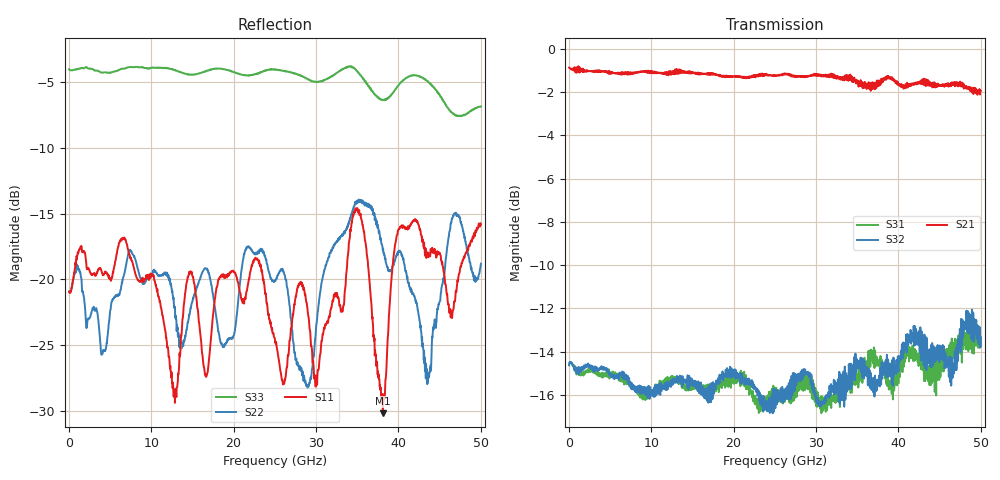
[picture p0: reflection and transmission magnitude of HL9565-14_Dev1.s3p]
! 1/5/2021 8:28:36 AM
! H:\PRODUCTION_DATA\TEMP_S3P.S3P
! CHANNEL.1
! TR.MEASUREMENT
! CORRECTED.DATA
# GHZ S RI R 50.0
! FREQ.GHZ  S11RE  S11IM  S12RE  S12IM  S13RE  S13IM
!  S21RE  S21IM  S22RE  S22IM  S23RE  S23IM
!  S31RE  S31IM  S32RE  S32IM  S33RE  S33IM
!; PortSelection: Port_123
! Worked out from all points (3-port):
!   1429 points, 35 MHz to 50.02 GHz, reference 50 ohm
!   strongest paths, dB at 35 MHz, 12.53 GHz, 25.02 GHz, 37.52 GHz, 50.02 GHz:
!     S21: -0.9, -1.1, -1.2, -1.6, -2.0
!     S32: -14.6, -15.5, -16.1, -15.3, -13.3
!     S31: -14.6, -15.5, -16.0, -14.4, -13.6
!   lowest |S11| = -30.2 dB at 38.12 GHz (marker M1), VSWR 1.06, Z = 53.1 + j0.699 ohm
!   |S11| at or under -10 dB: start of sweep to end of sweep
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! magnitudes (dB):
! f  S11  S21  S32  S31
! 35 MHz  -20.9  -0.9  -14.6  -14.6
! 25.02 GHz  -24.6  -1.2  -16.1  -16.0
! 29.05 GHz  -22.7  -1.3  -15.0  -15.0
! 30.1 GHz  -27.8  -1.2  -16.1  -15.8
! 35 GHz  -14.6  -1.6  -14.8  -15.1
! 38.12 GHz  -30.2  -1.5  -14.6  -14.5
! 40.18 GHz  -16.0  -1.7  -14.4  -14.8
! 43.58 GHz  -18.3  -1.5  -14.4  -14.7
! 46.69 GHz  -22.2  -1.7  -14.7  -13.6
! 50.02 GHz  -15.8  -2.0  -13.3  -13.6
